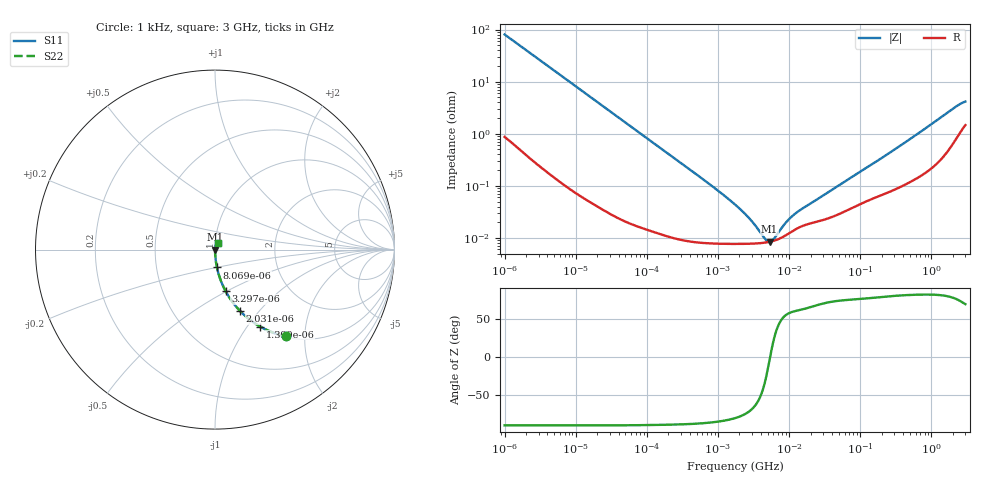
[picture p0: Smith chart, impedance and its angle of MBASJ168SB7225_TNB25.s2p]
! MBASJ168SB7225_TNB25  S-PARAMETER MODEL  ( Standard Model )
! Model Generated by TAIYO YUDEN Corporation (http://www.ty-top.com)
! Version 1.0
! TAIYO YUDEN Control No. 220601
! Copyright(c) 2015 TAIYO YUDEN CO.,LTD. All Rights Reserved.
! Product Description (link to TY-COMPAS)
! https://ds.yuden.co.jp/TYCOMPAS/or/detail?pn=MBASJ168SB7225KTNB25&u=M
! Products Name : Multilayer Ceramic Capacitors
! Characteristics :
!  Capacitance : 2.2 [uF] , Rated Voltage : 6.3 [V] , TCC : X7R
!  Case Size : 1.6 x 0.8 / 0.063 x 0.031 [mm/inch] , Thickness : 0.8 / 0.031 [mm/inch]
!  (Conditions: Temperature = 25 [degC] , DC Bias Voltage = 0 [V])
! External Node Assignments :
!  1  o---| |---o  2
! GND o---------o GND
! Frequency Range : 1kHz  -  3GHz  [ 401 STEP ]
# MHZ S RI R 50
! Freq[MHz].  S11 Real  S11 Imag  S21 Real  S21 Imag  S12 Real  S12 Imag  S22 Real  S22 Imag
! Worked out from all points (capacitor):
!   401 points, 1 kHz to 3 GHz, reference 50 ohm
!   read as one part in series: C = 1.98 uF near 1.077 kHz
!   lowest |Z| = 8.42 mohm at 5.301 MHz (marker M1)
!   series resonance near 5.395 MHz, so ESL is about 440 pH
!   S11 on the Smith chart (normalised r, x): 1 kHz: 1.02, -1.61; 1.399 kHz: 1.01, -1.15; 2.031 kHz: 1.01, -0.79; 3.297 kHz: 1.00, -0.49; 8.069 kHz: 1.00, -0.20; 3 GHz: 1.03, +0.08
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0.001  0.3931 -0.4831  0.6069 0.4831  0.6069 0.4831  0.3931 -0.4831
0.001399  0.2511 -0.4285  0.7489 0.4285  0.7489 0.4285  0.2511 -0.4285
0.002031  0.1388 -0.341  0.8612 0.341  0.8612 0.341  0.1388 -0.341
0.003297  0.0587 -0.2305  0.9413 0.2305  0.9413 0.2305  0.0587 -0.2305
0.008069  0.0109 -0.0995  0.9891 0.0995  0.9891 0.0995  0.0109 -0.0995
0.01216  0.00507 -0.0666  0.9949 0.0666  0.9949 0.0666  0.00507 -0.0666
0.033275  0.000874 -0.0246  0.9991 0.0246  0.9991 0.0246  0.000874 -0.0246
0.147855  0.000151 -0.00558  0.9998 0.00558  0.9998 0.00558  0.000151 -0.00558
0.762639  7.97e-05 -0.00107  0.9999 0.00107  0.9999 0.00107  7.97e-05 -0.00107
1.732051  7.69e-05 -0.000431  0.9999 0.000431  0.9999 0.000431  7.69e-05 -0.000431
2.812335  7.74e-05 -0.000216  0.9999 0.000216  0.9999 0.000216  7.74e-05 -0.000216
4.238263  8.02e-05 -7.59e-05  0.9999 7.59e-05  0.9999 7.59e-05  8.02e-05 -7.59e-05
4.739869  8.18e-05 -4.04e-05  0.9999 4.04e-05  0.9999 4.04e-05  8.18e-05 -4.04e-05
5.30084  8.41e-05 -5.43e-06  0.9999 5.43e-06  0.9999 5.43e-06  8.41e-05 -5.43e-06
6.387174  9e-05 5.29e-05  0.9999 -5.29e-05  0.9999 -5.29e-05  9e-05 5.29e-05
8.606987  0.000109 0.000148  0.9999 -0.000148  0.9999 -0.000148  0.000109 0.000148
10.76485  0.000131 0.000217  0.9999 -0.000217  0.9999 -0.000217  0.000131 0.000217
13.97519  0.00016 0.000296  0.9998 -0.000296  0.9998 -0.000296  0.00016 0.000296
21.06097  0.000194 0.000438  0.9998 -0.000438  0.9998 -0.000438  0.000194 0.000438
256.0921  0.000779 0.00419  0.9992 -0.00419  0.9992 -0.00419  0.000779 0.00419
2144.796  0.00827 0.0309  0.9917 -0.0309  0.9917 -0.0309  0.00827 0.0309
3000  0.0158 0.0376  0.9842 -0.0376  0.9842 -0.0376  0.0158 0.0376
